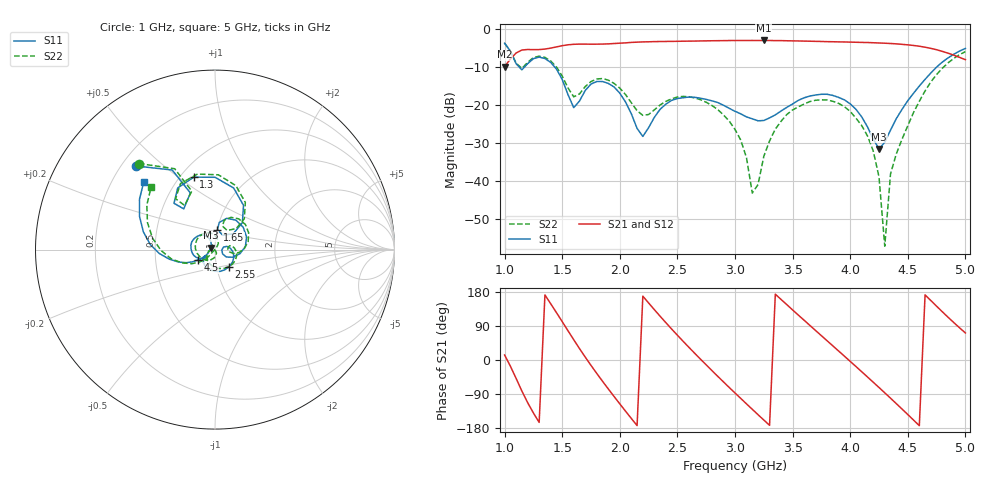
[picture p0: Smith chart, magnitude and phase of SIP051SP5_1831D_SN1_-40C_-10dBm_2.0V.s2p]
# GHz  S  dB  R  50
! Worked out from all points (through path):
!   81 points, 1 GHz to 5 GHz, reference 50 ohm
!   highest |S21| = -3.14 dB at 3.25 GHz (marker M1); lowest = -10.0 dB at 1 GHz (marker M2)
!   lowest |S11| = -31.7 dB at 4.25 GHz (marker M3), VSWR 1.05, Z = 47.6 + j0.949 ohm
!   |S11| at or under -10 dB: 1.123 GHz to 1.177 GHz (54.16 MHz wide, 4.71 % of centre); 1.431 GHz to 4.755 GHz (3.324 GHz wide, 107 % of centre)
!   |S22| runs from -57.3 to -3.9 dB; largest |S21 - S12| = 0.0021
!   S11 on the Smith chart (normalised r, x): 1 GHz: 0.26, +0.41; 1.3 GHz: 0.58, +0.57; 1.65 GHz: 1.00, +0.22; 2.55 GHz: 1.15, -0.22; 4.5 GHz: 0.82, -0.10; 5 GHz: 0.33, +0.36
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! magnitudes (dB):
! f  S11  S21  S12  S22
! 1 GHz  -3.9  -10.0  -10.0  -3.9
! 1.15 GHz  -10.9  -5.7  -5.7  -10.5
! 1.3 GHz  -7.5  -5.5  -5.5  -7.3
! 1.65 GHz  -19.1  -4.1  -4.1  -17.2
! 1.7 GHz  -16.3  -4.1  -4.1  -15.3
! 1.95 GHz  -15.4  -4.0  -4.0  -14.4
! 2.2 GHz  -28.4  -3.5  -3.5  -22.8
! 2.35 GHz  -21.2  -3.4  -3.4  -20.1
! 2.55 GHz  -18.2  -3.3  -3.3  -17.9
! 3 GHz  -21.8  -3.2  -3.2  -26.6
! 3.1 GHz  -23.3  -3.2  -3.1  -34.0
! 3.15 GHz  -23.8  -3.1  -3.1  -43.3
! 3.25 GHz  -24.2  -3.1  -3.1  -33.6
! 3.45 GHz  -20.7  -3.2  -3.2  -22.6
! 3.7 GHz  -17.5  -3.4  -3.4  -18.9
! 4.05 GHz  -21.3  -3.6  -3.6  -23.6
! 4.25 GHz  -31.7  -3.8  -3.8  -39.0
! 4.3 GHz  -29.9  -3.9  -3.9  -57.3
! 4.35 GHz  -26.7  -3.9  -4.0  -38.3
! 4.5 GHz  -19.0  -4.3  -4.3  -25.6
! 4.75 GHz  -10.1  -5.6  -5.6  -12.1
! 5 GHz  -5.2  -8.2  -8.2  -6.1
